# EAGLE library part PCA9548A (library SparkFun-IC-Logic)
Texas Instruments PCA9548A - I2C Multiplexer The PCA9548A device has eight bidirectional translating switches that can be controlled through the I2C bus. The SCL/SDA upstream pair fans out to eight downstream pairs, or channels. Any individual SCn/SDn channel or combination of channels can be selected, determined by the contents of the programmable control register. These downstream channels can be used to resolve I2C slave address conflicts.
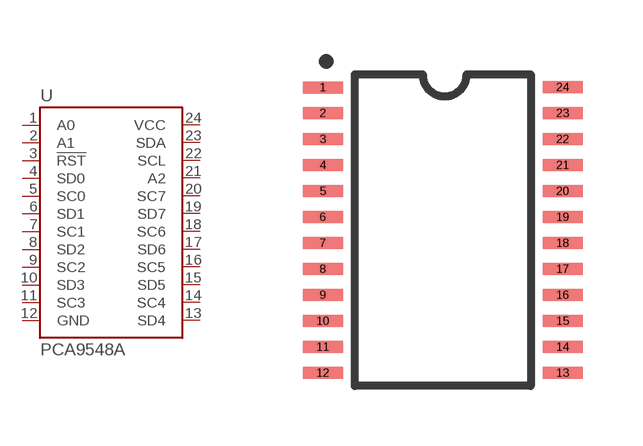
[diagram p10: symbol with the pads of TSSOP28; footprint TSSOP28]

Designator prefix U

## PCA9548A (PROD_ID: IC-13948)  [TSSOP28]
1  A0
2  A1
3  !RST
4  SD0
5  SC0
6  SD1
7  SC1
8  SD2
9  SC2
10  SD3
11  SC3
12  GND
13  SD4
14  SC4
15  SD5
16  SC5
17  SD6
18  SC6
19  SD7
20  SC7
21  A2
22  SCL
23  SDA
24  VCC

## Footprint TSSOP28 (pad centres in mm)
TSSOP-28 - [Package Short Description] Specifications: Pin count: 28 Pin pitch: .65 mm Area: 6.6 mm x 7.9 mm Datasheet referenced for footprint
smd 1 x 0.3: 1 -3,3.57; 2 -3,2.925; 3 -3,2.275; 4 -3,1.625; 5 -3,0.975; 6 -3,0.325; 7 -3,-0.325; 8 -3,-0.975; 9 -3,-1.625; 10 -3,-2.275; 11 -3,-2.925; 12 -3,-3.575; 13 3,-3.575; 14 3,-2.925; 15 3,-2.275; 16 3,-1.625; 17 3,-0.975; 18 3,-0.325; 19 3,0.325; 20 3,0.975; 21 3,1.625; 22 3,2.275; 23 3,2.925; 24 3,3.575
